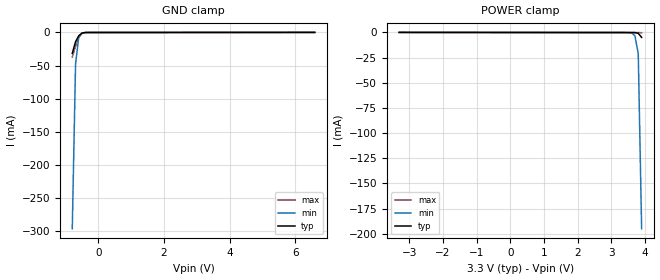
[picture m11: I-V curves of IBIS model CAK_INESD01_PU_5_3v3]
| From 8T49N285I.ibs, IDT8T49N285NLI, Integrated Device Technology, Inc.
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[Model] CAK_INESD01_PU_5_3v3
Model_type   Input
Polarity   Non-Inverting
Vinl = 0.8V
Vinh = 2.0V
|   typ   min   max
C_comp   2pF   1.5pF   2.5pF
|   typ   min   max
[Voltage range]   3.3V   3.135V   3.465V
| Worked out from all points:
|   GND clamp passes 1 mA (typ) near -0.50 V on its own axis
[GND_clamp]
|Voltage   I (typ)   I (min)   I (max)
|Note, modeling breaks down at 250mA and above.  This is well beyond the functional   |
|operating range of the device.  Should this scenario occur, catastrophic failure and   |
|possible damage to the device and/or board is of higher concern than the I-V curve   |
|behavior.  The IBIS checker will flag currents in excess of 10A with warnings.  Lines   |
|with currents in excess of 0.35 A have been commented out.  The points still remain|
|available to the user if the user desires to use them.   |
|-3.30000e+00   -9.36890e+00   -7.41800e+00   -1.15554e+01
|-3.20000e+00   -8.98680e+00   -7.13126e+00   -1.10682e+01
|-3.10000e+00   -8.60472e+00   -6.84459e+00   -1.05810e+01
|-3.00000e+00   -8.22265e+00   -6.55802e+00   -1.00938e+01
|-2.90000e+00   -7.84061e+00   -6.27153e+00   -9.60652e+00
|-2.80000e+00   -7.45860e+00   -5.98514e+00   -9.11925e+00
|-2.70000e+00   -7.07663e+00   -5.69886e+00   -8.63197e+00
|-2.60000e+00   -6.69471e+00   -5.41269e+00   -8.14469e+00
|-2.50000e+00   -6.31284e+00   -5.12664e+00   -7.65742e+00
|-2.40000e+00   -5.93104e+00   -4.84073e+00   -7.17015e+00
|-2.30000e+00   -5.54933e+00   -4.55496e+00   -6.68291e+00
|-2.20000e+00   -5.16771e+00   -4.26934e+00   -6.19571e+00
|-2.10000e+00   -4.78621e+00   -3.98390e+00   -5.70857e+00
|-2.00000e+00   -4.40484e+00   -3.69864e+00   -5.22150e+00
|-1.90000e+00   -4.02364e+00   -3.41358e+00   -4.73454e+00
|-1.80000e+00   -3.64262e+00   -3.12873e+00   -4.24771e+00
|-1.70000e+00   -3.26181e+00   -2.84411e+00   -3.76103e+00
|-1.60000e+00   -2.88126e+00   -2.55973e+00   -3.27453e+00
|-1.50000e+00   -2.50099e+00   -2.27561e+00   -2.78824e+00
|-1.40000e+00   -2.12106e+00   -1.99177e+00   -2.30221e+00
|-1.30000e+00   -1.74151e+00   -1.70822e+00   -1.81651e+00
|-1.20000e+00   -1.36238e+00   -1.42497e+00   -1.33120e+00
|-1.10000e+00   -9.83731e-01   -1.14207e+00   -8.46369e-01
|-1.00000e+00   -6.05610e-01   -8.59548e-01   -3.62110e-01
|-9.00000e-01   -2.28086e-01   -5.77564e-01   -5.71865e-02
-800mV    -31.58mA   -296.4mA   -37.13mA
-700mV    -14.02mA   -47.95mA   -20.86mA
-600mV    -4.892mA   -5.99mA    -7.57mA
-500mV    -845.2uA   -939.7uA   -1.201mA
-300mV    -73.38uA   -66.8uA    -87.49uA
6.6V      65.77uA    60.51uA    72.18uA
[Power_clamp]
|Voltage   I (typ)   I (min)   I (max)
|Note, modeling breaks down at 250mA and above.  This is well beyond the functional   |
|operating range of the device.  Should this scenario occur, catastrophic failure and   |
|possible damage to the device and/or board is of higher concern than the I-V curve   |
|behavior.  The IBIS checker will flag currents in excess of 10A with warnings.  Lines   |
|with currents in excess of 0.35 A have been commented out.  The points still remain|
|available to the user if the user desires to use them.   |
-3.3V     65.77uA    57.64uA    75.99uA
3.5V      -69.75uA   -98.2uA    -80.55uA
3.6V      -73.38uA   -468.3uA   -82.85uA
3.7V      -124.1uA   -3.105mA   -85.19uA
3.8V      -845.2uA   -21.26mA   -91.47uA
3.9V      -4.892mA   -195mA     -262.6uA
